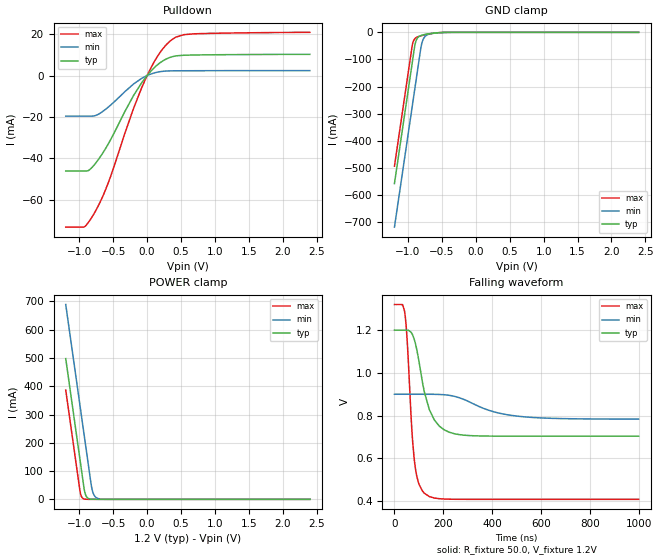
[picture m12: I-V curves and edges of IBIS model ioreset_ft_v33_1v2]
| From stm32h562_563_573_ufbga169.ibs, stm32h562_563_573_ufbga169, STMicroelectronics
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[Model]   ioreset_ft_v33_1v2
Model_type I/O_open_drain
Polarity   Inverting
Enable   Active-Low
| CAP_THRESHOLD on pad IOFT is "UDTCAPC" :
| Rising=20.0% of vddiom   Falling=80.0% of vddiom
| C_comp min and max val. don't necessarily correlate with the min and max pvt
| but are the smallest and greatest pad capacitance found.
| var   typ   min   max
C_comp   2.84130pF  2.76215pF  2.88040pF
|C_comp_pulldown   2.84130pF  2.76215pF  2.88040pF
Vinl = 450.0mV
Vinh = 660.0mV
Vmeas = 600.0mV   | Reference voltage for timing measurements
Cref  = 50.0pF   | Timing specification test load capacitance value
Rref  = 1.0MOhm   | Timing specification test load resistance value
Vref  = 660.0mV   | Timing specification test load voltage
[Model Spec]
| TIME_THRESHOLD on pin ZIV33M is "CMOS" :
| Rising=40.0% of vddiom   Falling=60.0% of vddiom
Vinl 443.80000mV 340.80000mV 485.80000mV
Vinh 727.20000mV 529.20000mV 807.20000mV
| variable   typ   min   max
[Temperature Range] 25.0 125.0 -40.0
| variable   typ   min   max
[Voltage Range] 1.2V 900.0mV 1.32V
| variable   typ   min   max
[POWER Clamp Reference] 1.2V 900.0mV 1.32V
| variable   typ   min   max
[GND Clamp Reference] 0V 0V 0V
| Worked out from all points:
|   slope of the pulldown table from 0 to 0.18 V, typ, clamps not added: 30.6 ohm
|   GND clamp passes 1 mA (typ) near -0.52 V on its own axis
|   POWER clamp passes 1 mA (typ) near -0.84 V on its own axis
|   falling waveform, R_fixture 50.0, V_fixture 1.2V: 20-80 % time 60.6ns typ, 166ns min, 28.8ns max; typ from 1.2 V to 0.704 V
[POWER Clamp]
-1.2V     497.8mA    689.2mA    386.5mA
-990mV    140.8mA    332.2mA    29.53mA
-980mV    123.8mA    315.2mA    17.95mA
-960mV    89.81mA    281.2mA    6.634mA
-930mV    38.81mA    230.2mA    1.49mA
-900mV    12.07mA    179.2mA    334.8uA
-870mV    3.756mA    128.2mA    75.22uA
-820mV    536.4uA    44.98mA    6.245uA
-790mV    166.9uA    18.76mA    1.403uA
-750mV    35.18uA    5.847mA    191.7nA
-590mV    69.59nA    55.16uA    84.18pA
2.4V      0A         0A         0A
[GND Clamp]
-1.2V     -558.2mA   -719mA     -494.1mA
-940mV    -116.2mA   -277mA     -52.06mA
-930mV    -99.18mA   -260mA     -39.94mA
-900mV    -49.1mA    -209mA     -23.75mA
-880mV    -30.13mA   -175mA     -19.59mA
-850mV    -17.82mA   -124mA     -16.09mA
-810mV    -11.73mA   -56.78mA   -12.9mA
-780mV    -9.44mA    -28.21mA   -10.91mA
-740mV    -7.285mA   -13.16mA   -8.565mA
-640mV    -3.567mA   -4.168mA   -3.948mA
-390mV    -79.81uA   -270.3uA   -28.73uA
2.4V      233.9pA    35.97nA    60.57pA
| variable   typ   min   max
[Pullup Reference] 1.2V 900.0mV 1.32V
| variable   typ   min   max
[Pulldown Reference] 0V 0V 0V
[Pulldown]
-1.2V     -46.17mA   -19.62mA   -73.27mA
-930mV    -46.17mA   -19.62mA   -73.18mA
-860mV    -45.79mA   -19.62mA   -70.72mA
-770mV    -42.8mA    -19.41mA   -66.04mA
-570mV    -32.88mA   -15.18mA   -51.58mA
-200mV    -9.658mA   -4.083mA   -15.89mA
-80mV     -3.488mA   -1.363mA   -5.887mA
140mV     4.817mA    1.546mA    8.585mA
350mV     8.893mA    2.257mA    16.93mA
540mV     9.805mA    2.305mA    19.74mA
670mV     9.907mA    2.32mA     20.12mA
2.4V      10.24mA    2.38mA     20.88mA
[Ramp]
dV/dt_r 297.02691mV/1.29501ns 69.92336mV/4.07755ns 547.69816mV/634.55203ps
dV/dt_f 297.80521mV/59.252ns 69.83691mV/166.01957ns 547.13931mV/28.75647ns
R_load = 50.0
| Removed startup time: 0s 0s 0s  .
| Removed end time: 349.99us.
[Falling Waveform]
R_fixture   = 50.0
V_fixture   = 1.2V
V_fixture_min = 900.0mV
V_fixture_max = 1.32V
0s        1.2V       900mV      1.32V
41.35ns   1.2V       900mV      1.288V
51.3ns    1.2V       900mV      1.165V
70.8ns    1.185V     900mV      741.6mV
81.55ns   1.155V     900mV      590.4mV
122.3ns   911mV      900mV      436.6mV
163.1ns   779.9mV    899.7mV    414.3mV
244.6ns   715.4mV    890.5mV    408.4mV
489.2ns   703.7mV    799.4mV    408.1mV
998.7ns   703.7mV    783.6mV    408.1mV
